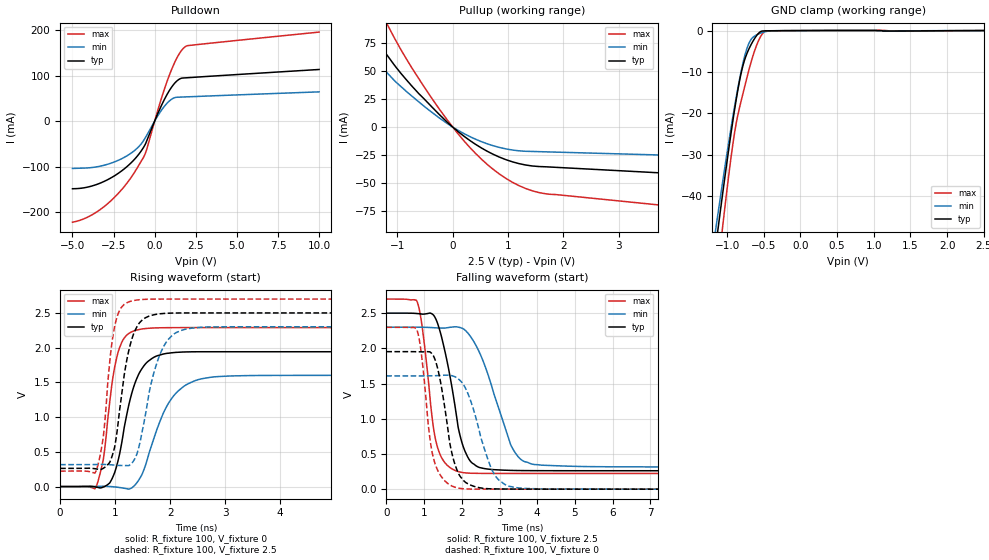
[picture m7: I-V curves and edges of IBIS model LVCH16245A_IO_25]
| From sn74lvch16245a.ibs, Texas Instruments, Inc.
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[Model]   LVCH16245A_IO_25
Model_type  3-state
Enable   Active-Low
Vref =   0
Rref =   500
Cref =   30p
Vmeas =   1.25
| variable   typ   min   max
C_comp   4.60pF   4.14pF   5.47pF
| C_pullup   5.74pF   3.90pF   8.57pF
| C_pulldown   7.30pF   4.83pF   9.26pF
| C_tri-state   4.60pF   4.14pF   5.47pF
[Temperature Range]   40   100   -40
| Ambient temperature   25   85   -40
[Voltage range]   2.5   2.3   2.7
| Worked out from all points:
|   slope of the pulldown table from 0 to 0.375 V, typ, clamps not added: 11.9 ohm
|   slope of the pullup table from 0 to 0.375 V, typ, clamps not added: 26.5 ohm
|   GND clamp passes 1 mA (typ) near -0.59 V on its own axis
|   rising waveform, R_fixture 100, V_fixture 0: 20-80 % time 335ps typ, 482ps min, 224ps max; typ from 0 V to 1.94 V
|   falling waveform, R_fixture 100, V_fixture 2.5: 20-80 % time 466ps typ, 746ps min, 325ps max; typ from 2.5 V to 0.262 V
|   rising waveform, R_fixture 100, V_fixture 2.5: 20-80 % time 258ps typ, 343ps min, 183ps max; typ from 0.262 V to 2.5 V
|   falling waveform, R_fixture 100, V_fixture 0: 20-80 % time 374ps typ, 547ps min, 293ps max; typ from 1.95 V to 0 V
[GND Clamp]
| LVCH16245A_IO_25
|   Voltage   I(typ)   I(min)   I(max)
-5V       -657.8mA   -597.1mA   -758.7mA
-1.165V   -53.45mA   -49.09mA   -63.7mA
-1.13V    -48.64mA   -44.79mA   -58.1mA
-1.095V   -43.89mA   -40.55mA   -52.57mA
-1.065V   -39.88mA   -36.97mA   -47.9mA
-900mV    -19.27mA   -18.49mA   -24.83mA
-785mV    -8.516mA   -7.918mA   -15.26mA
-725mV    -5.32mA    -4.071mA   -11.01mA
-670mV    -3.271mA   -2.057mA   -7.407mA
-565mV    -538.3uA   -766.3uA   -2.183mA
-485mV    -73.08uA   -294.4uA   -219.6uA
2.5V      13.87pA    76.94nA    -1.18nA
[Pulldown]
| LVCH16245A_IO_25
|   Voltage   I(typ)   I(min)   I(max)
-5V       -148.4mA   -103.9mA   -221.8mA
-4.05V    -144.6mA   -102.7mA   -210.3mA
-3.075V   -132.4mA   -96.92mA   -187.6mA
-2.11V    -112mA     -84.36mA   -154.5mA
-1.27V    -85.53mA   -65.87mA   -114.9mA
-850mV    -67.03mA   -51.33mA   -89.83mA
-540mV    -48.37mA   -34.68mA   -68.09mA
230mV     19.76mA    13.93mA    28.68mA
750mV     58.22mA    39.1mA     86.73mA
1.33V     87.32mA    52.22mA    137mA
1.83V     94.73mA    52.98mA    162.4mA
10V       113.2mA    64.1mA     195.3mA
[Pullup]
| LVCH16245A_IO_25
|   Voltage   I(typ)   I(min)   I(max)
-5V       239.2mA    81.99mA    492.7mA
-4.68V    312.1mA    90.43mA    464.8mA
-1.855V   114.9mA    88.16mA    163.1mA
-1.56V    92.11mA    70.47mA    130.2mA
-1.19V    64.67mA    48.88mA    92.59mA
-830mV    41.95mA    31.63mA    60.41mA
-400mV    19.25mA    14.1mA     27.37mA
310mV     -12mA      -8.479mA   -18.25mA
960mV     -29.11mA   -19.47mA   -45.88mA
1.56V     -35.28mA   -21.93mA   -58.6mA
7.4V      -50.58mA   -29.97mA   -88.15mA
10V       -57.52mA   -33.56mA   -101.4mA
[Ramp]
| LVCH16245A_IO_25
| variable   typ   min   max
dV/dt_r   1.18/3.42E-10   0.98/5.02E-10   1.39/2.29E-10
dV/dt_f   1.34/4.88E-10   1.19/7.50E-10   1.49/3.28E-10
R_load = 100
[Rising Waveform]
| LVCH16245A_IO_25
R_fixture =   100
C_fixture =   0
L_fixture =   0
V_fixture =   0
V_fixture_min = 0
V_fixture_max = 0
|   Time   V(typ)   V(min)   V(max)
0s        -22.65uV   -31.11uV   -11.46uV
645ps     -5.581mV   1.432mV    -14.61mV
785ps     -7.111mV   4.883mV    393.4mV
900ps     51.46mV    925.9uV    1.209V
1.135ns   704mV      -20.4mV    2.101V
1.355ns   1.479V     17.82mV    2.245V
1.64ns    1.828V     541.9mV    2.281V
2.14ns    1.934V     1.373V     2.289V
3.09ns    1.941V     1.593V     2.289V
49.99ns   1.942V     1.602V     2.289V
[Falling Waveform]
| LVCH16245A_IO_25
R_fixture =   100
C_fixture =   0
L_fixture =   0
V_fixture =   2.5
V_fixture_min = 2.3
V_fixture_max = 2.7
|   Time   V(typ)   V(min)   V(max)
0s        2.5V       2.3V       2.7V
825ps     2.494V     2.3V       2.651V
975ps     2.486V     2.3V       2.206V
1.285ns   2.445V     2.292V     758.7mV
1.56ns    1.943V     2.289V     369.8mV
2.1ns     521.3mV    2.252V     231mV
2.555ns   297.6mV    1.833V     224mV
3.36ns    266mV      565.8mV    222.8mV
4.12ns    262.5mV    340.7mV    222.6mV
49.99ns   261.8mV    316.2mV    222.6mV
[Rising Waveform]
| LVCH16245A_IO_25
R_fixture =   100
C_fixture =   0
L_fixture =   0
V_fixture =   2.5
V_fixture_min = 2.3
V_fixture_max = 2.7
|   Time   V(typ)   V(min)   V(max)
0s        261.7mV    316.1mV    222.6mV
650ps     255.1mV    317.1mV    221.8mV
785ps     263.3mV    318.8mV    722.2mV
900ps     346.6mV    314.5mV    1.787V
1.09ns    1.157V     304mV      2.551V
1.275ns   2.046V     316.9mV    2.667V
1.5ns     2.404V     828.8mV    2.694V
1.915ns   2.494V     2.064V     2.7V
2.665ns   2.5V       2.298V     2.7V
49.99ns   2.5V       2.3V       2.7V
[Falling Waveform]
| LVCH16245A_IO_25
R_fixture =   100
C_fixture =   0
L_fixture =   0
V_fixture =   0
V_fixture_min = 0
V_fixture_max = 0
|   Time   V(typ)   V(min)   V(max)
0s        1.953V     1.609V     2.299V
810ps     1.952V     1.609V     2.264V
925ps     1.95V      1.609V     1.94V
1.25ns    1.892V     1.611V     440.4mV
1.435ns   1.529V     1.615V     196.8mV
1.755ns   473.1mV    1.609V     40.87mV
2.055ns   118.1mV    1.478V     5.145mV
2.85ns    4.253mV    222.8mV    500.7uV
3.66ns    657.2uV    10.72mV    91.34uV
49.99ns   8.613uV    47.57uV    348.6nV
